(* Logix 5000 AddOnInstructionDefinition export POINT_ADD; software revision 30.00 *)

TYPE POINT :   // A point on an Edwards-curve represented in extended homogeneous coordinates
STRUCT
   X : DINT[22];
   Y : DINT[22];
   Z : DINT[22];
   T : DINT[22];
END_STRUCT
END_TYPE

ADD_ON_INSTRUCTION B256_ADD   (* revision 1.0 20170916, vendor Kenneth A. Fischer *)
// c3=c1+c2 with no reduction
// Revision note:
// Rev1.0: 20170916 - Initial Release
VAR_IN_OUT
   Inp_C1 : DINT[22]; {required}
   Inp_C2 : DINT[22]; {required}
   Out_C3 : DINT[22]; {required}
END_VAR
VAR
   i : INT;
END_VAR

ROUTINE Logic   (* ladder *)
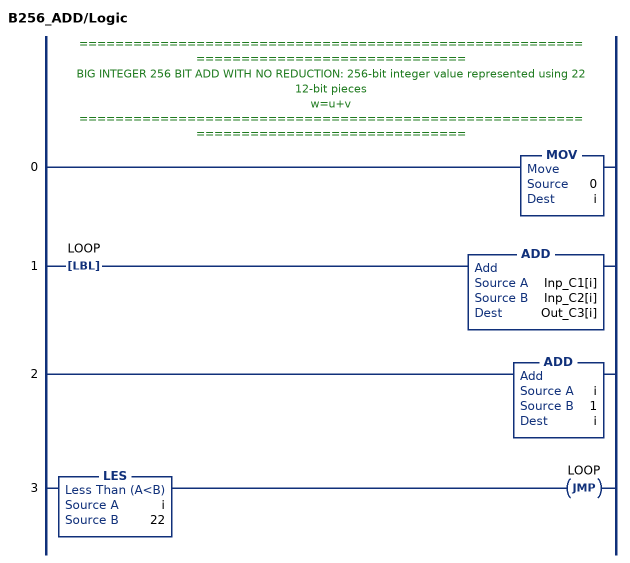
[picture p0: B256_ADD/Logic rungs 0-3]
   // ======================================================================================
   // BIG INTEGER 256 BIT ADD WITH NO REDUCTION: 256-bit integer value represented using 22 12-bit pieces
   // w=u+v
   // ======================================================================================
   0: MOV(0,i);
   1: LBL(LOOP)ADD(Inp_C1[i],Inp_C2[i],Out_C3[i]);
   2: ADD(i,1,i);
   3: LES(i,22)JMP(LOOP);
END_ROUTINE
END_ADD_ON_INSTRUCTION

ADD_ON_INSTRUCTION D_SHR   (* revision 1.0 20170524, vendor Kenneth A. Fischer *)
// DINT bit shift right of the 32-bit argument Inp_A by Inp_B bits with paddding by zeros on the right
// Revision note:
// Rev1.0: 20170524 - Initial Release
VAR_IN_OUT
   Inp_A : DINT; {required}   // 64-bit Integer to be right circular rotated
END_VAR
VAR_INPUT
   Inp_B : INT; {required}   // Number of bits to shift
END_VAR
VAR_IN_OUT
   Out : DINT; {required}   // Result
END_VAR
VAR
   BSR_Cntrl : CONTROL := (LEN := 32);
   ONS : BOOL;
   Source_Bit : BOOL;
   Wrk_InpA : DINT[2];
END_VAR

ROUTINE Logic   (* ladder *)
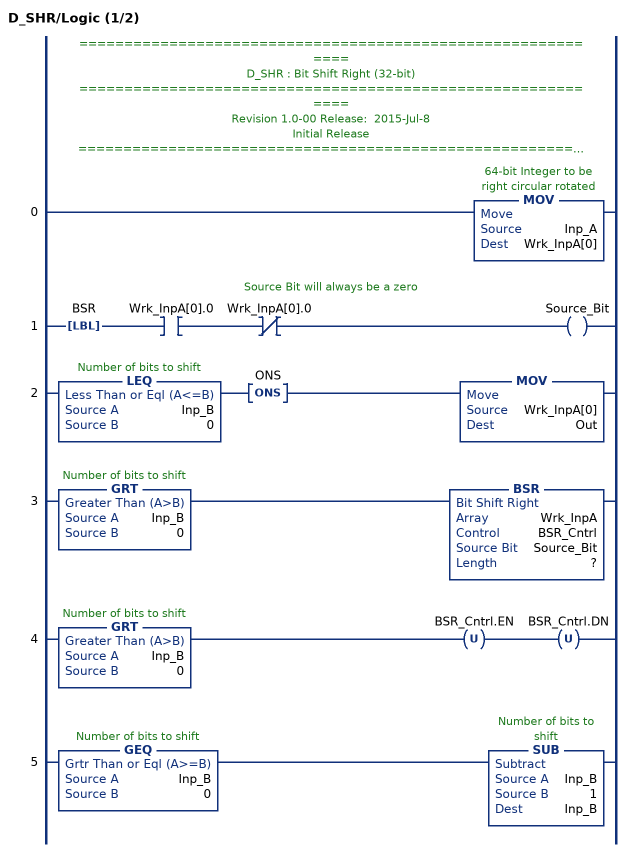
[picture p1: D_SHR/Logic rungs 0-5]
   // ============================================================
   // D_SHR : Bit Shift Right (32-bit)
   // ============================================================
   // Revision 1.0-00 Release:  2015-Jul-8
   // Initial Release
   // ============================================================
   // Performs a right bit shift of the 32-bit argument Inp_A by the
   // number of bits defined in the 16-bit argument Inp_B, with padding by zeros.
   0: MOV(Inp_A,Wrk_InpA[0]);
   // Source Bit will always be a zero
   1: LBL(BSR)XIC(Wrk_InpA[0].0)XIO(Wrk_InpA[0].0)OTE(Source_Bit);
   2: LEQ(Inp_B,0)ONS(ONS)MOV(Wrk_InpA[0],Out);
   3: GRT(Inp_B,0)BSR(Wrk_InpA,BSR_Cntrl,Source_Bit,?);
   4: GRT(Inp_B,0)OTU(BSR_Cntrl.EN)OTU(BSR_Cntrl.DN);
   5: GEQ(Inp_B,0)SUB(Inp_B,1,Inp_B);
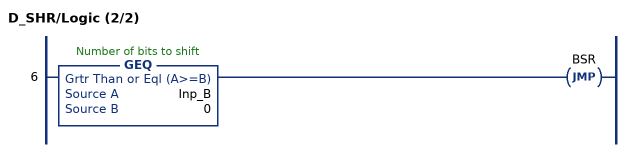
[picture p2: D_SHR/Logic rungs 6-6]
   6: GEQ(Inp_B,0)JMP(BSR);
END_ROUTINE
END_ADD_ON_INSTRUCTION

ADD_ON_INSTRUCTION B256_NRED   (* revision 1.0 20170916, vendor Kenneth A. Fischer *)
// Reduce 256-bit integer stored in 22 pieces by propagating carries
// Revision note:
// Rev1.0: 20170916 - Initial Release
VAR_IN_OUT
   Inp_C : DINT[22]; {required}
END_VAR
VAR
   D_SHR : D_SHR;
   temp : DINT;
   i : INT;
END_VAR

ROUTINE Logic   (* ladder *)
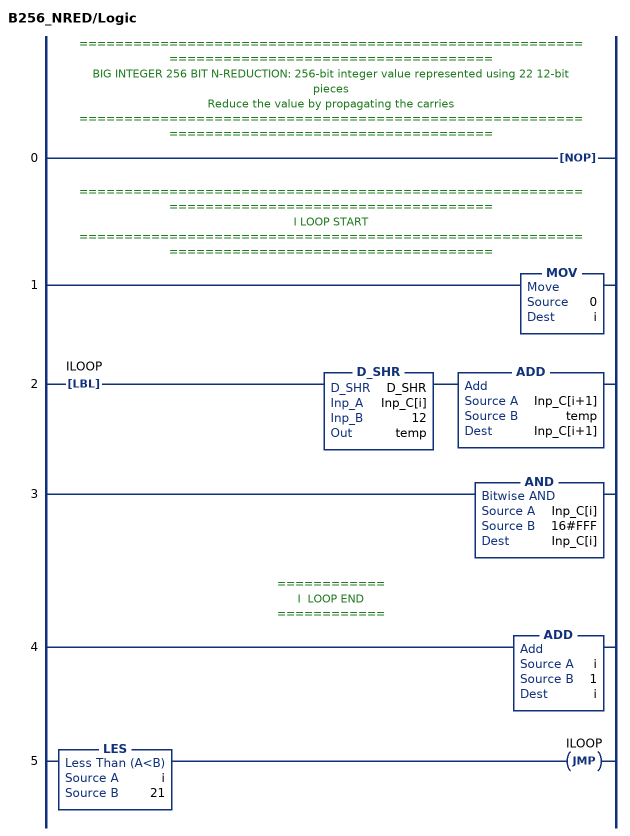
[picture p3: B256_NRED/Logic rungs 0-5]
   // ============================================================================================
   // BIG INTEGER 256 BIT N-REDUCTION: 256-bit integer value represented using 22 12-bit pieces
   // Reduce the value by propagating the carries
   // ============================================================================================
   0: NOP();
   // ============================================================================================
   // I LOOP START
   // ============================================================================================
   1: MOV(0,i);
   2: LBL(ILOOP)D_SHR(D_SHR,Inp_C[i],12,temp)ADD(Inp_C[i+1],temp,Inp_C[i+1]);
   3: AND(Inp_C[i],16#FFF,Inp_C[i]);
   // ============
   // I  LOOP END
   // ============
   4: ADD(i,1,i);
   5: LES(i,21)JMP(ILOOP);
END_ROUTINE
END_ADD_ON_INSTRUCTION

ADD_ON_INSTRUCTION B256_SUB   (* revision 1.0 20170916, vendor Kenneth A. Fischer *)
// c3=c1-c2 with reduction
// Revision note:
// Rev1.0: 20170916 - Initial Release
VAR_IN_OUT
   Inp_C1 : DINT[22]; {required}
   Inp_C2 : DINT[22]; {required}
   Out_C3 : DINT[22]; {required}
END_VAR
VAR
   B256_ADD : B256_ADD;
   B256_NRED : B256_NRED;
   temp : DINT;
   i : INT;
END_VAR

ROUTINE Logic   (* ladder *)
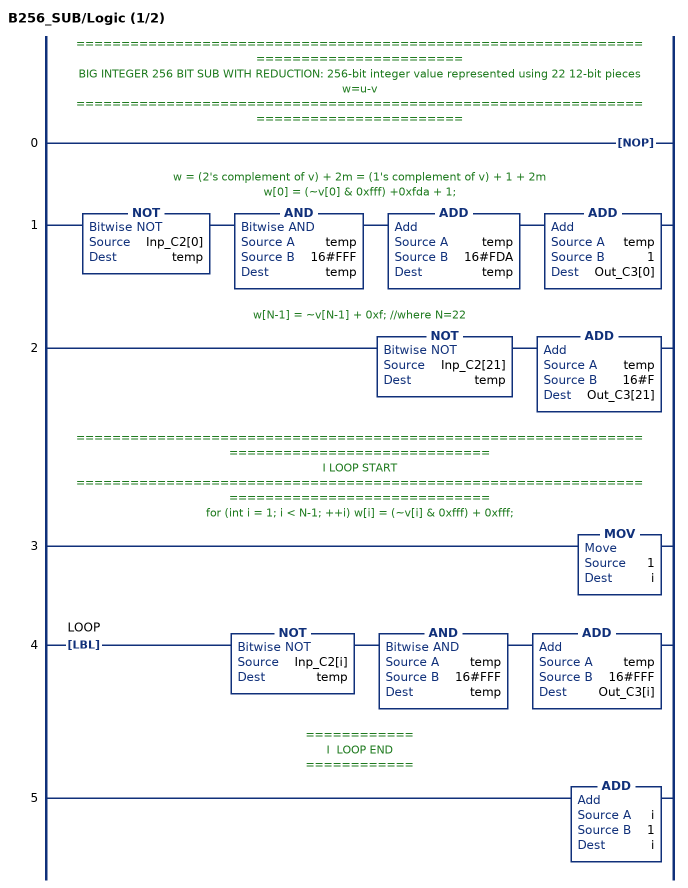
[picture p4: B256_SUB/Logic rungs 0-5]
   // ======================================================================================
   // BIG INTEGER 256 BIT SUB WITH REDUCTION: 256-bit integer value represented using 22 12-bit pieces
   //  w=u-v
   // ======================================================================================
   0: NOP();
   // w = (2's complement of v) + 2m = (1's complement of v) + 1 + 2m
   // w[0] = (~v[0] & 0xfff) +0xfda + 1;
   1: NOT(Inp_C2[0],temp)AND(temp,16#FFF,temp)ADD(temp,16#FDA,temp)ADD(temp,1,Out_C3[0]);
   // w[N-1] = ~v[N-1] + 0xf; //where N=22
   2: NOT(Inp_C2[21],temp)ADD(temp,16#F,Out_C3[21]);
   // ============================================================================================
   // I LOOP START
   // ============================================================================================
   // for (int i = 1; i < N-1; ++i) w[i] = (~v[i] & 0xfff) + 0xfff;
   3: MOV(1,i);
   4: LBL(LOOP)NOT(Inp_C2[i],temp)AND(temp,16#FFF,temp)ADD(temp,16#FFF,Out_C3[i]);
   // ============
   // I  LOOP END
   // ============
   5: ADD(i,1,i);
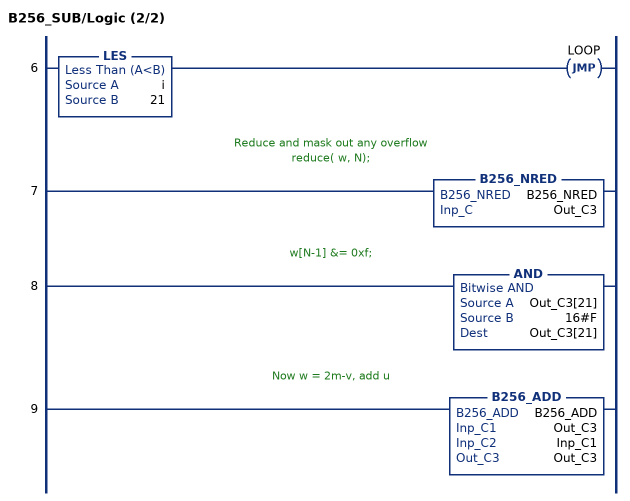
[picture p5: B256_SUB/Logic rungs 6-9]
   6: LES(i,21)JMP(LOOP);
   // Reduce and mask out any overflow
   // reduce( w, N);
   7: B256_NRED(B256_NRED,Out_C3);
   // w[N-1] &= 0xf;
   8: AND(Out_C3[21],16#F,Out_C3[21]);
   // Now w = 2m-v, add u
   9: B256_ADD(B256_ADD,Out_C3,Inp_C1,Out_C3);
END_ROUTINE
END_ADD_ON_INSTRUCTION

ADD_ON_INSTRUCTION B256_FRED   (* revision 1.0 20170916, vendor Kenneth A. Fischer *)
// fast_reduce:  reduce by propagating the carries starting at a particular offset and stoping once the carry becomes zero
// Revision note:
// Rev1.0: 20170916 - Initial Release
VAR_IN_OUT
   Inp_C : DINT[22]; {required}
END_VAR
VAR_INPUT
   Inp_offset : INT; {required}
END_VAR
VAR
   i : INT;
   carry : DINT;
   D_SHR : D_SHR;
END_VAR

ROUTINE Logic   (* ladder *)
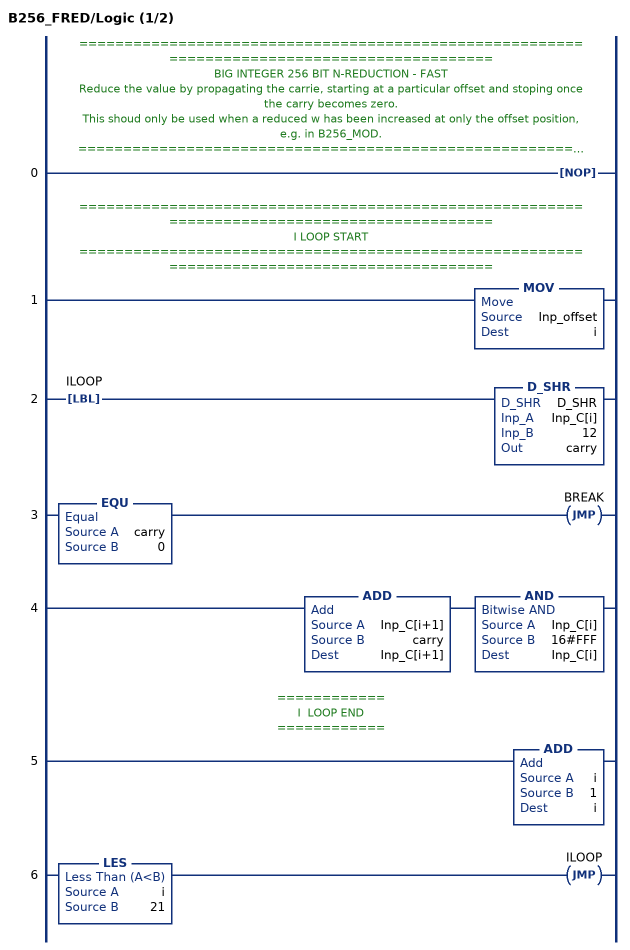
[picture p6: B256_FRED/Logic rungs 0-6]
   // ============================================================================================
   // BIG INTEGER 256 BIT N-REDUCTION - FAST
   // Reduce the value by propagating the carrie, starting at a particular offset and stoping once the carry becomes zero.
   // This shoud only be used when a reduced w has been increased at only the offset position, e.g. in B256_MOD.
   // ============================================================================================
   0: NOP();
   // ============================================================================================
   // I LOOP START
   // ============================================================================================
   1: MOV(Inp_offset,i);
   2: LBL(ILOOP)D_SHR(D_SHR,Inp_C[i],12,carry);
   3: EQU(carry,0)JMP(BREAK);
   4: ADD(Inp_C[i+1],carry,Inp_C[i+1])AND(Inp_C[i],16#FFF,Inp_C[i]);
   // ============
   // I  LOOP END
   // ============
   5: ADD(i,1,i);
   6: LES(i,21)JMP(ILOOP);
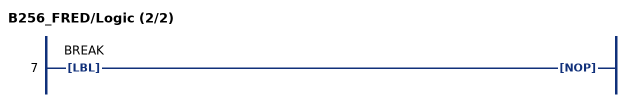
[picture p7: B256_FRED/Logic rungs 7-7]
   7: LBL(BREAK)NOP();
END_ROUTINE
END_ADD_ON_INSTRUCTION

ADD_ON_INSTRUCTION D_SHL   (* revision 1.0 20170524, vendor Kenneth A. Fischer *)
// DINT bit shift left of the 32-bit argument Inp_A by Inp_B bits with paddding by zeros on the right
// Revision note:
// Rev1.0: 20170524 - Initial Release
VAR_IN_OUT
   Inp_A : DINT; {required}   // 64-bit Integer to be right circular rotated
END_VAR
VAR_INPUT
   Inp_B : INT; {required}   // Number of bits to shift
END_VAR
VAR_IN_OUT
   Out : DINT; {required}   // Result
END_VAR
VAR
   Wrk_InpA : DINT[2];
   Source_Bit : BOOL;
   ONS : BOOL;
   BSL_Cntrl : CONTROL := (LEN := 32);
END_VAR

ROUTINE Logic   (* ladder *)
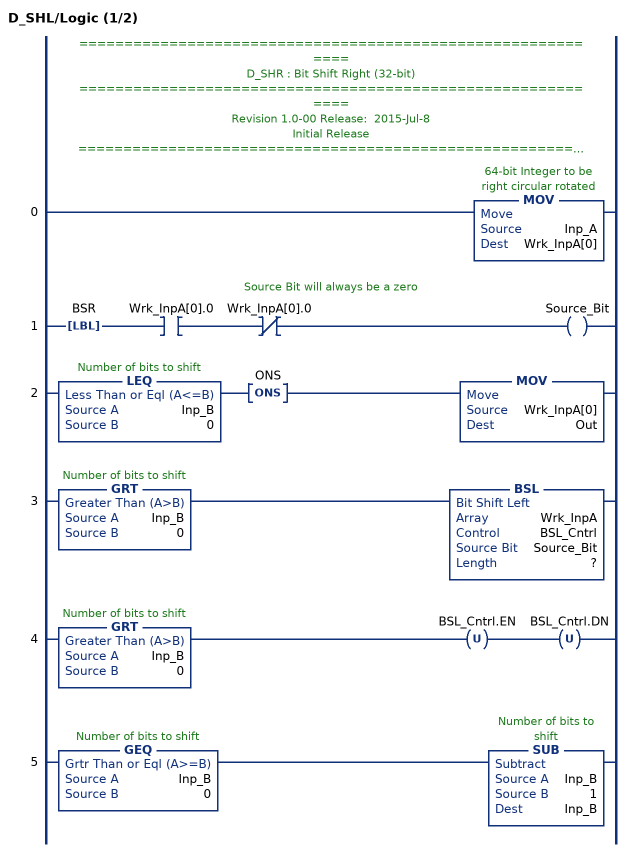
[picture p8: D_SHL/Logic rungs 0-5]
   // ============================================================
   // D_SHR : Bit Shift Right (32-bit)
   // ============================================================
   // Revision 1.0-00 Release:  2015-Jul-8
   // Initial Release
   // ============================================================
   // Performs a left bit shift of the 32-bit argument Inp_A by the
   // number of bits defined in the 16-bit argument Inp_B, with padding by zeros.
   0: MOV(Inp_A,Wrk_InpA[0]);
   // Source Bit will always be a zero
   1: LBL(BSR)XIC(Wrk_InpA[0].0)XIO(Wrk_InpA[0].0)OTE(Source_Bit);
   2: LEQ(Inp_B,0)ONS(ONS)MOV(Wrk_InpA[0],Out);
   3: GRT(Inp_B,0)BSL(Wrk_InpA,BSL_Cntrl,Source_Bit,?);
   4: GRT(Inp_B,0)OTU(BSL_Cntrl.EN)OTU(BSL_Cntrl.DN);
   5: GEQ(Inp_B,0)SUB(Inp_B,1,Inp_B);
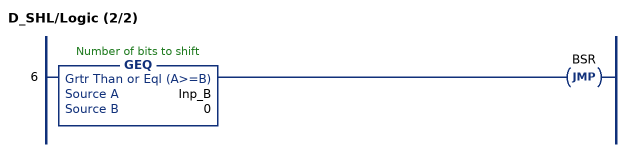
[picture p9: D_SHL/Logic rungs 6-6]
   6: GEQ(Inp_B,0)JMP(BSR);
END_ROUTINE
END_ADD_ON_INSTRUCTION

ADD_ON_INSTRUCTION B256_MOD   (* revision 1.0 20170916, vendor Kenneth A. Fischer *)
// c = d mod (2^255 - 19)
// Revision note:
// Rev1.0: 20170916 - Initial Release
VAR_IN_OUT
   Inp_D : DINT[43]; {required}
   Out_C : DINT[22]; {required}
END_VAR
VAR
   B256_NRED : B256_NRED;
   D_SHL : D_SHL;
   D_SHR : D_SHR;
   i : INT;
   t : DINT;
   temp : DINT;
   temp2 : DINT;
   B256_FRED : B256_FRED;
   offset : DINT;
END_VAR

ROUTINE Logic   (* ladder *)
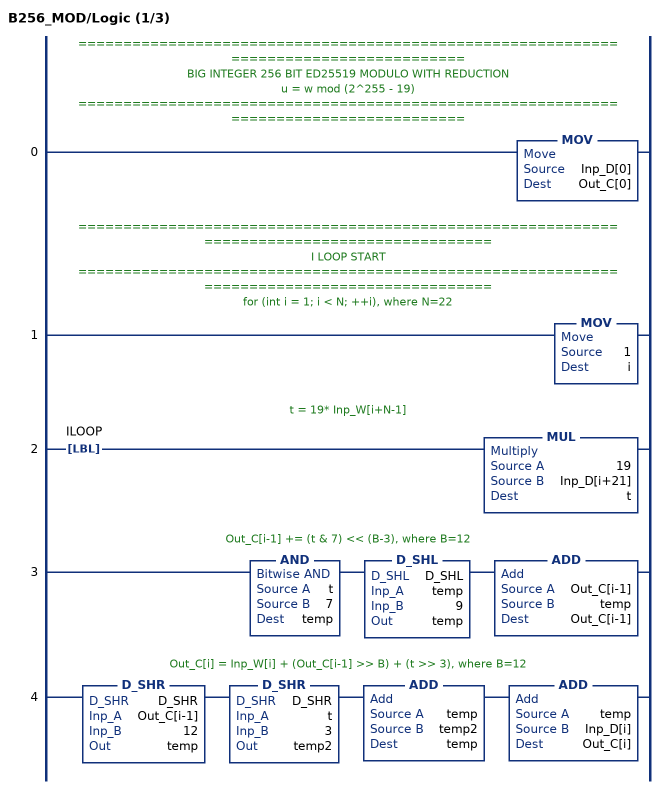
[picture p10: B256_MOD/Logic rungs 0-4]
   // ======================================================================================
   // BIG INTEGER 256 BIT ED25519 MODULO WITH REDUCTION
   //  u = w mod (2^255 - 19)
   // ======================================================================================
   0: MOV(Inp_D[0],Out_C[0]);
   // ============================================================================================
   // I LOOP START
   // ============================================================================================
   // for (int i = 1; i < N; ++i), where N=22
   1: MOV(1,i);
   // t = 19* Inp_W[i+N-1]
   2: LBL(ILOOP)MUL(19,Inp_D[i+21],t);
   // Out_C[i-1] += (t & 7) << (B-3), where B=12
   3: AND(t,7,temp)D_SHL(D_SHL,temp,9,temp)ADD(Out_C[i-1],temp,Out_C[i-1]);
   // Out_C[i] = Inp_W[i] + (Out_C[i-1] >> B) + (t >> 3), where B=12
   4: D_SHR(D_SHR,Out_C[i-1],12,temp)D_SHR(D_SHR,t,3,temp2)ADD(temp,temp2,temp)ADD(temp,Inp_D[i],Out_C[i]);
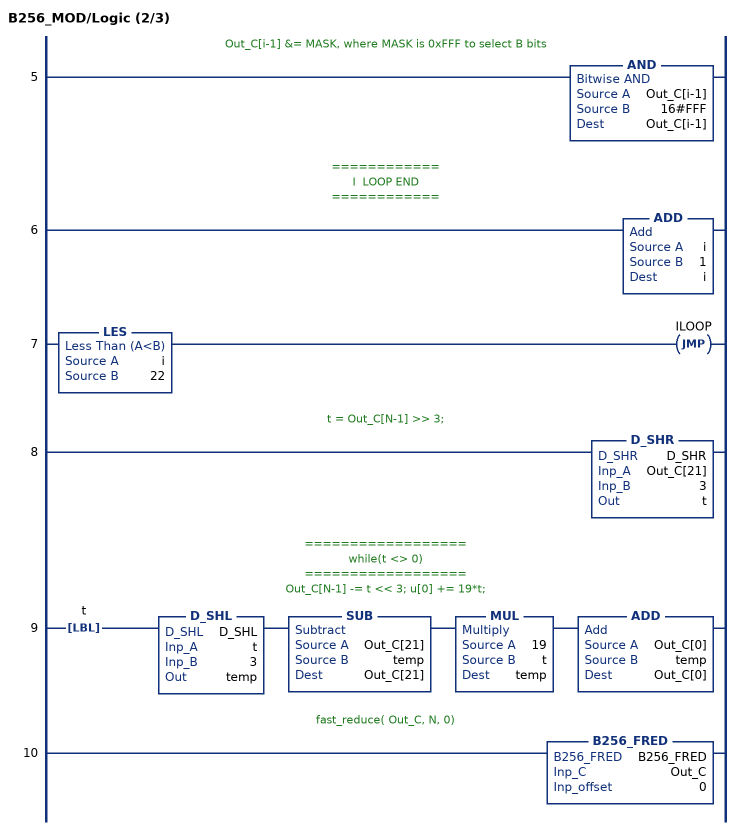
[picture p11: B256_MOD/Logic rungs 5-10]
   // Out_C[i-1] &= MASK, where MASK is 0xFFF to select B bits
   5: AND(Out_C[i-1],16#FFF,Out_C[i-1]);
   // ============
   // I  LOOP END
   // ============
   6: ADD(i,1,i);
   7: LES(i,22)JMP(ILOOP);
   // t = Out_C[N-1] >> 3;
   8: D_SHR(D_SHR,Out_C[21],3,t);
   // ==================
   // while(t <> 0)
   // ==================
   // Out_C[N-1] -= t << 3; u[0] += 19*t;
   9: LBL(t)D_SHL(D_SHL,t,3,temp)SUB(Out_C[21],temp,Out_C[21])MUL(19,t,temp)ADD(Out_C[0],temp,Out_C[0]);
   // fast_reduce( Out_C, N, 0)
   10: B256_FRED(B256_FRED,Out_C,0);
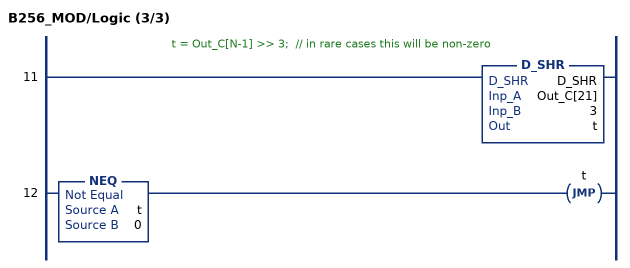
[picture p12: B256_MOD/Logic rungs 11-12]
   // t = Out_C[N-1] >> 3;  // in rare cases this will be non-zero
   11: D_SHR(D_SHR,Out_C[21],3,t);
   12: NEQ(t,0)JMP(t);
END_ROUTINE
END_ADD_ON_INSTRUCTION

ADD_ON_INSTRUCTION B256_NNRED   (* revision 1.0 20170916, vendor Kenneth A. Fischer *)
// Reduce 256-bit integer stored in 43 pieces by propagating carries
// Revision note:
// Rev1.0: 20170916 - Initial Release
VAR_IN_OUT
   Inp_D : DINT[43]; {required}
END_VAR
VAR
   temp : DINT;
   i : INT;
   D_SHR : D_SHR;
END_VAR

ROUTINE Logic   (* ladder *)
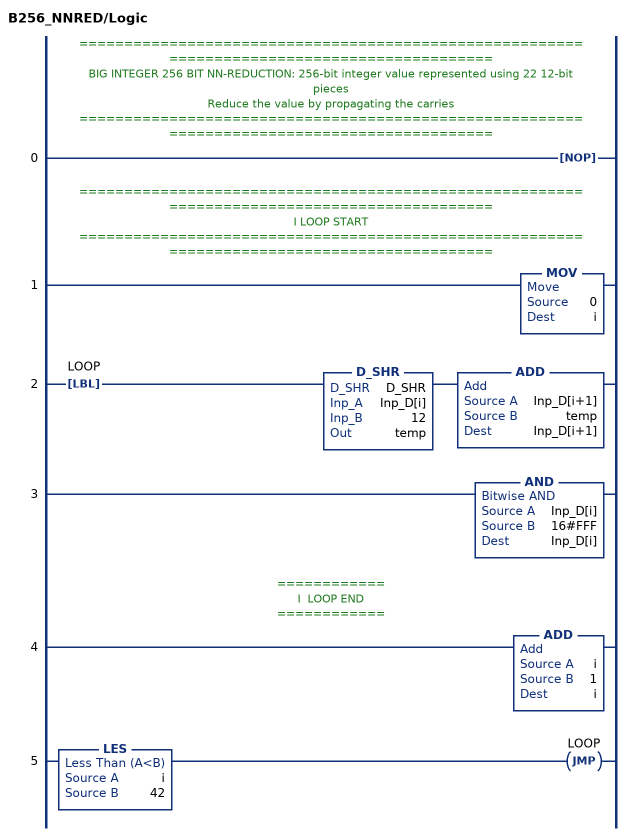
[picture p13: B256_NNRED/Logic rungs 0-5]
   // ============================================================================================
   // BIG INTEGER 256 BIT NN-REDUCTION: 256-bit integer value represented using 22 12-bit pieces
   // Reduce the value by propagating the carries
   // ============================================================================================
   0: NOP();
   // ============================================================================================
   // I LOOP START
   // ============================================================================================
   1: MOV(0,i);
   2: LBL(LOOP)D_SHR(D_SHR,Inp_D[i],12,temp)ADD(Inp_D[i+1],temp,Inp_D[i+1]);
   3: AND(Inp_D[i],16#FFF,Inp_D[i]);
   // ============
   // I  LOOP END
   // ============
   4: ADD(i,1,i);
   5: LES(i,42)JMP(LOOP);
END_ROUTINE
END_ADD_ON_INSTRUCTION

ADD_ON_INSTRUCTION B256_MUL   (* revision 1.0 20170916, vendor Kenneth A. Fischer *)
// c3 = c1*c2 with reduction and mod
// Revision note:
// Rev1.0: 20170916 - Initial Release
VAR_IN_OUT
   Temp_D : DINT[43]; {required}
   Inp_C1 : DINT[22]; {required}
   Inp_C2 : DINT[22]; {required}
   Out_C3 : DINT[22]; {required}
END_VAR
VAR
   B256_MOD : B256_MOD;
   B256_NNRED : B256_NNRED;
   i : INT;
   j : INT;
   mul_temp : DINT;
END_VAR

ROUTINE Logic   (* ladder *)
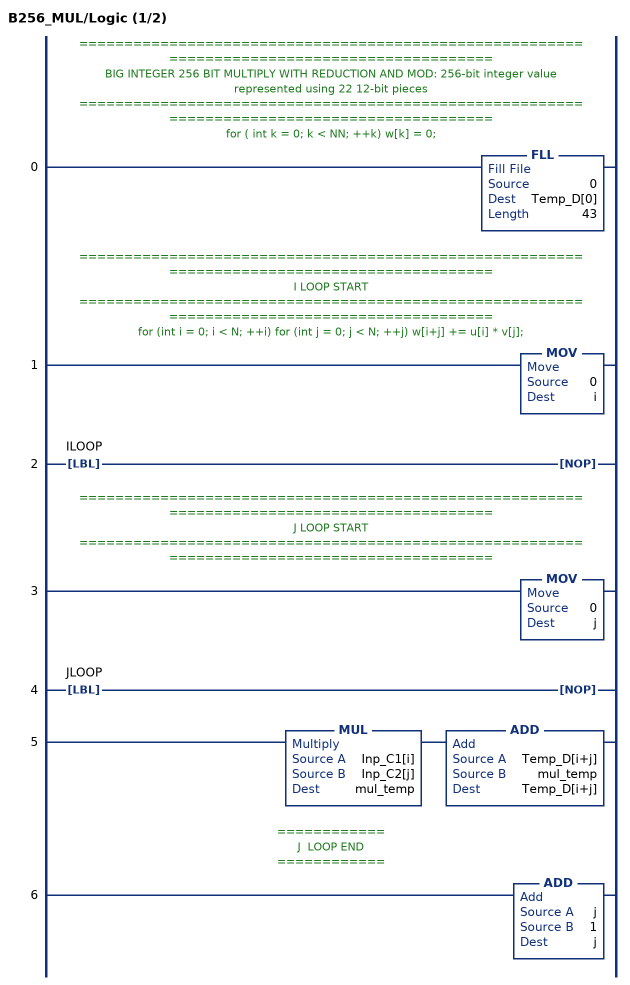
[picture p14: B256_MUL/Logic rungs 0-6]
   // ============================================================================================
   // BIG INTEGER 256 BIT MULTIPLY WITH REDUCTION AND MOD: 256-bit integer value represented using 22 12-bit pieces
   // ============================================================================================
   // for ( int k = 0; k < NN; ++k) w[k] = 0;
   0: FLL(0,Temp_D[0],43);
   // ============================================================================================
   // I LOOP START
   // ============================================================================================
   // for (int i = 0; i < N; ++i) for (int j = 0; j < N; ++j) w[i+j] += u[i] * v[j];
   1: MOV(0,i);
   2: LBL(ILOOP)NOP();
   // ============================================================================================
   // J LOOP START
   // ============================================================================================
   3: MOV(0,j);
   4: LBL(JLOOP)NOP();
   5: MUL(Inp_C1[i],Inp_C2[j],mul_temp)ADD(Temp_D[i+j],mul_temp,Temp_D[i+j]);
   // ============
   // J  LOOP END
   // ============
   6: ADD(j,1,j);
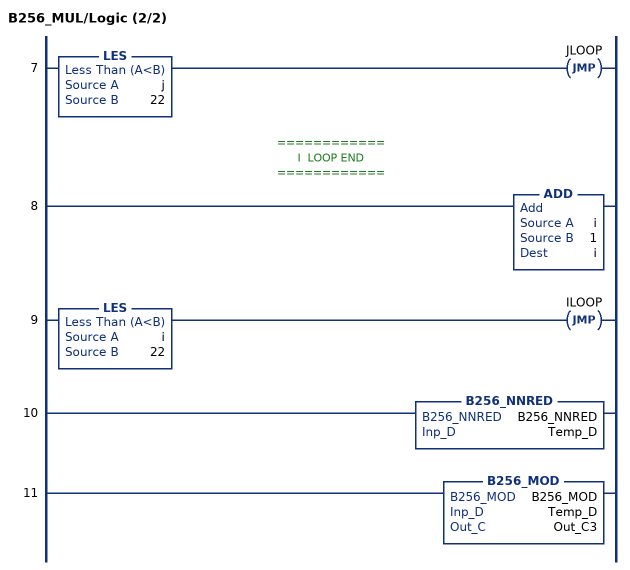
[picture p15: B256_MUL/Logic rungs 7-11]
   7: LES(j,22)JMP(JLOOP);
   // ============
   // I  LOOP END
   // ============
   8: ADD(i,1,i);
   9: LES(i,22)JMP(ILOOP);
   10: B256_NNRED(B256_NNRED,Temp_D);
   11: B256_MOD(B256_MOD,Temp_D,Out_C3);
END_ROUTINE
END_ADD_ON_INSTRUCTION

ADD_ON_INSTRUCTION B256_MUL2   (* revision 1.0 20170916, vendor Kenneth A. Fischer *)
// c3= 2*c1*c2 with reduction and mod
// Revision note:
// Rev1.0: 20170916 - Initial Release
VAR_IN_OUT
   Temp_D : DINT[43]; {required}
   Inp_C1 : DINT[22]; {required}
   Inp_C2 : DINT[22]; {required}
   Out_C3 : DINT[22]; {required}
END_VAR
VAR
   B256_NNRED : B256_NNRED;
   i : INT;
   j : INT;
   mul_temp : DINT;
   B256_MOD : B256_MOD;
   t : DINT;
END_VAR

ROUTINE Logic   (* ladder *)
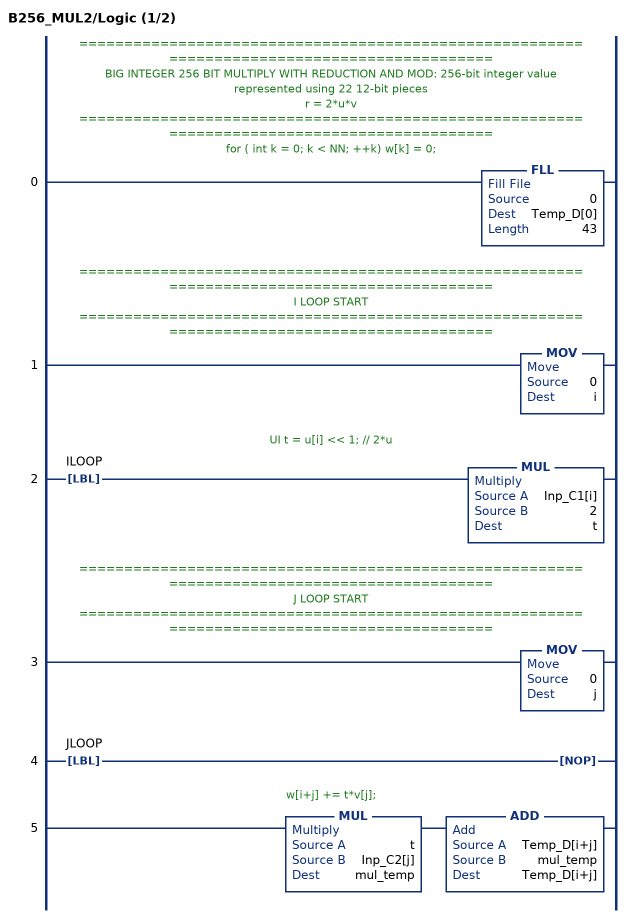
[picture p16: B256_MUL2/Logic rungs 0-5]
   // ============================================================================================
   // BIG INTEGER 256 BIT MULTIPLY WITH REDUCTION AND MOD: 256-bit integer value represented using 22 12-bit pieces
   // r = 2*u*v
   // ============================================================================================
   // for ( int k = 0; k < NN; ++k) w[k] = 0;
   0: FLL(0,Temp_D[0],43);
   // ============================================================================================
   // I LOOP START
   // ============================================================================================
   1: MOV(0,i);
   // UI t = u[i] << 1; // 2*u
   2: LBL(ILOOP)MUL(Inp_C1[i],2,t);
   // ============================================================================================
   // J LOOP START
   // ============================================================================================
   3: MOV(0,j);
   4: LBL(JLOOP)NOP();
   // w[i+j] += t*v[j];
   5: MUL(t,Inp_C2[j],mul_temp)ADD(Temp_D[i+j],mul_temp,Temp_D[i+j]);
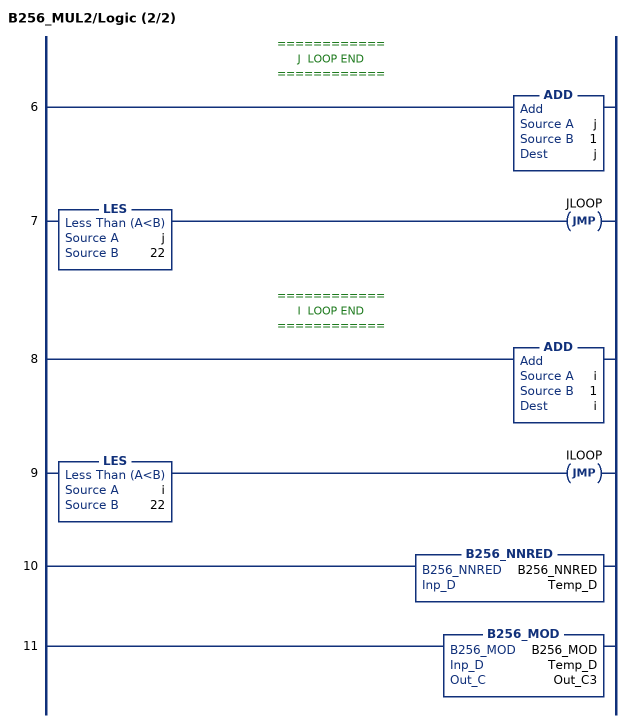
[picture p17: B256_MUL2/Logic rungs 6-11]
   // ============
   // J  LOOP END
   // ============
   6: ADD(j,1,j);
   7: LES(j,22)JMP(JLOOP);
   // ============
   // I  LOOP END
   // ============
   8: ADD(i,1,i);
   9: LES(i,22)JMP(ILOOP);
   10: B256_NNRED(B256_NNRED,Temp_D);
   11: B256_MOD(B256_MOD,Temp_D,Out_C3);
END_ROUTINE
END_ADD_ON_INSTRUCTION

ADD_ON_INSTRUCTION POINT_ADD   (* revision 1.0 20170916, vendor Kenneth A. Fischer *)
// Point Add:
// p3 = p1 + p2
// Requires POINT UDT
// Revision note:
// Rev1.0: 20170916 - Initial Release
VAR_IN_OUT
   Temp_C1 : DINT[22]; {required}   // A
   Temp_C2 : DINT[22]; {required}   // B
   Temp_C3 : DINT[22]; {required}   // C
   Temp_C4 : DINT[22]; {required}   // D
   Temp_C5 : DINT[22]; {required}   // E
   Temp_C6 : DINT[22]; {required}   // F
   Temp_C7 : DINT[22]; {required}   // G
   Temp_C8 : DINT[22]; {required}   // H
   Temp_C9 : DINT[22]; {required}   // R
   Temp_C10 : DINT[22]; {required}   // S
   Temp_D : DINT[43]; {required}   // W
   Inp_P1 : POINT; {required}
   Inp_P2 : POINT; {required}
   Out_P3 : POINT; {required}
END_VAR
VAR
   B256_SUB : B256_SUB;
   B256_ADD : B256_ADD;
   B256_MUL : B256_MUL;
   B256_MUL2 : B256_MUL2;
END_VAR

ROUTINE Logic   (* ladder *)
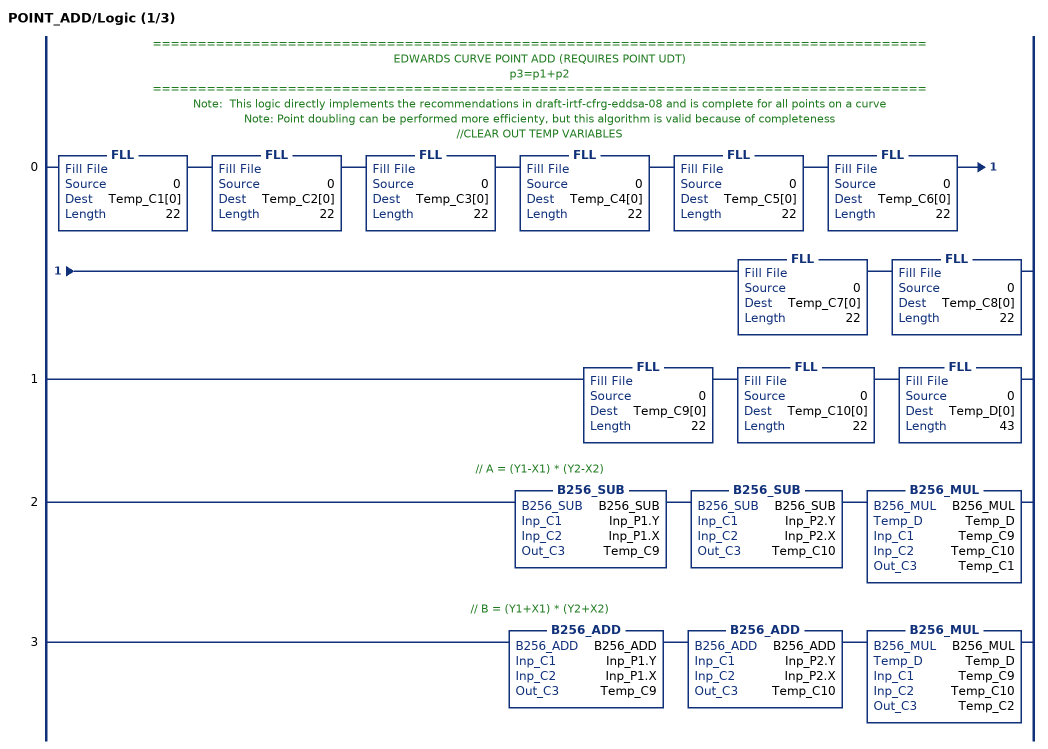
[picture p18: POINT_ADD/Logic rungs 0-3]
   // ======================================================================================
   // EDWARDS CURVE POINT ADD (REQUIRES POINT UDT)
   // p3=p1+p2
   // ======================================================================================
   // Note:  This logic directly implements the recommendations in draft-irtf-cfrg-eddsa-08 and is complete for all points on a curve
   // Note: Point doubling can be performed more efficienty, but this algorithm is valid because of completeness
   // //CLEAR OUT TEMP VARIABLES
   0: FLL(0,Temp_C1[0],22)FLL(0,Temp_C2[0],22)FLL(0,Temp_C3[0],22)FLL(0,Temp_C4[0],22)FLL(0,Temp_C5[0],22)FLL(0,Temp_C6[0],22)FLL(0,Temp_C7[0],22)FLL(0,Temp_C8[0],22);
   1: FLL(0,Temp_C9[0],22)FLL(0,Temp_C10[0],22)FLL(0,Temp_D[0],43);
   // // A = (Y1-X1) * (Y2-X2)
   2: B256_SUB(B256_SUB,Inp_P1.Y,Inp_P1.X,Temp_C9)B256_SUB(B256_SUB,Inp_P2.Y,Inp_P2.X,Temp_C10)B256_MUL(B256_MUL,Temp_D,Temp_C9,Temp_C10,Temp_C1);
   // // B = (Y1+X1) * (Y2+X2)
   3: B256_ADD(B256_ADD,Inp_P1.Y,Inp_P1.X,Temp_C9)B256_ADD(B256_ADD,Inp_P2.Y,Inp_P2.X,Temp_C10)B256_MUL(B256_MUL,Temp_D,Temp_C9,Temp_C10,Temp_C2);
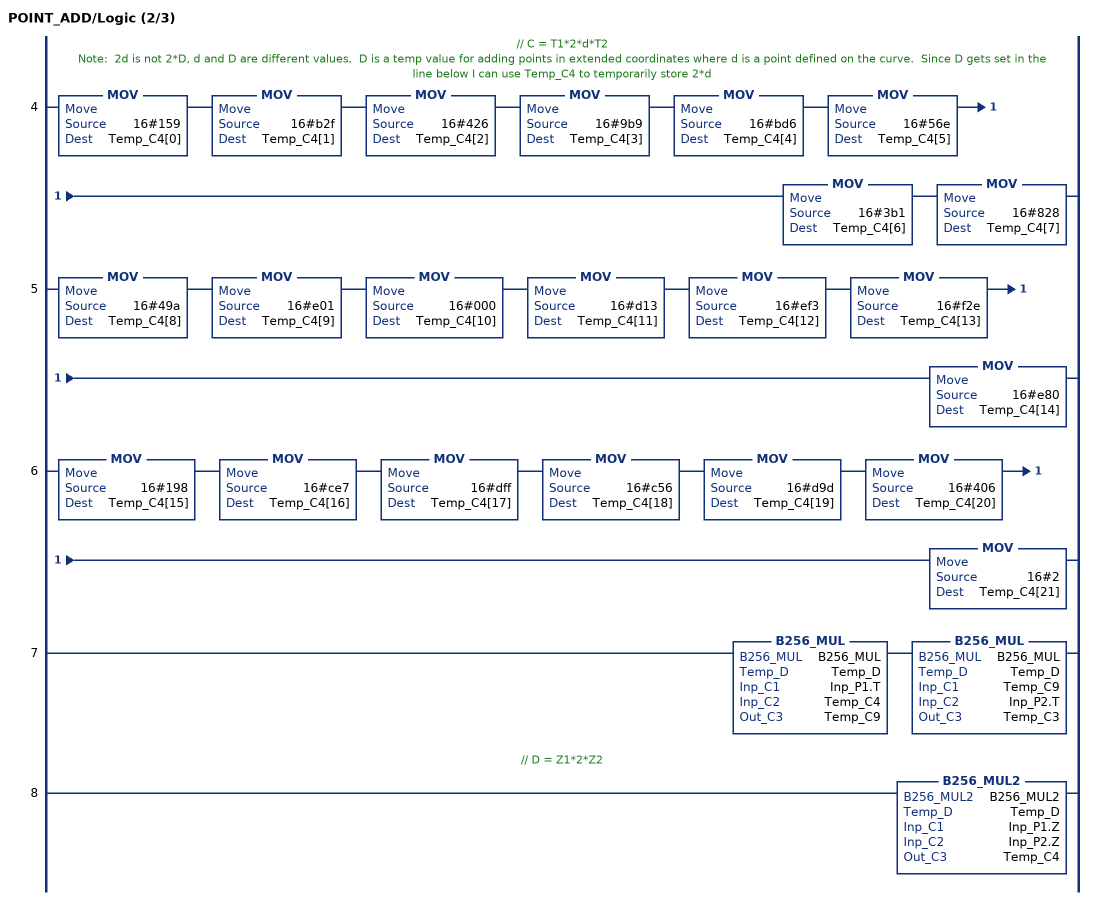
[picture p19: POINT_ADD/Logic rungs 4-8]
   // // C = T1*2*d*T2
   // Note:  2d is not 2*D, d and D are different values.  D is a temp value for adding points in extended coordinates where d is a point defined on the curve.  Since D gets set in the line below I can use Temp_C4 to temporarily store 2*d
   4: MOV(16#159,Temp_C4[0])MOV(16#b2f,Temp_C4[1])MOV(16#426,Temp_C4[2])MOV(16#9b9,Temp_C4[3])MOV(16#bd6,Temp_C4[4])MOV(16#56e,Temp_C4[5])MOV(16#3b1,Temp_C4[6])MOV(16#828,Temp_C4[7]);
   5: MOV(16#49a,Temp_C4[8])MOV(16#e01,Temp_C4[9])MOV(16#000,Temp_C4[10])MOV(16#d13,Temp_C4[11])MOV(16#ef3,Temp_C4[12])MOV(16#f2e,Temp_C4[13])MOV(16#e80,Temp_C4[14]);
   6: MOV(16#198,Temp_C4[15])MOV(16#ce7,Temp_C4[16])MOV(16#dff,Temp_C4[17])MOV(16#c56,Temp_C4[18])MOV(16#d9d,Temp_C4[19])MOV(16#406,Temp_C4[20])MOV(16#2,Temp_C4[21]);
   7: B256_MUL(B256_MUL,Temp_D,Inp_P1.T,Temp_C4,Temp_C9)B256_MUL(B256_MUL,Temp_D,Temp_C9,Inp_P2.T,Temp_C3);
   // // D = Z1*2*Z2
   8: B256_MUL2(B256_MUL2,Temp_D,Inp_P1.Z,Inp_P2.Z,Temp_C4);
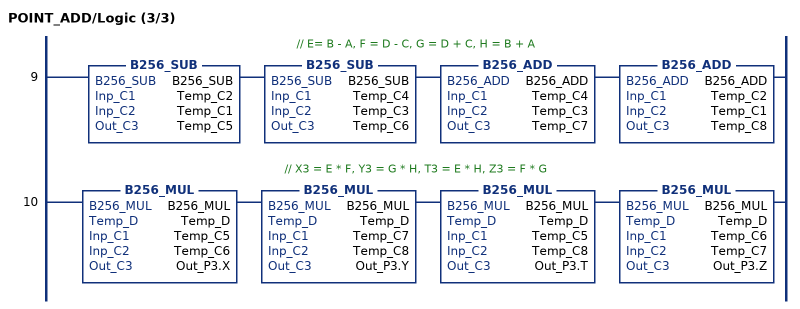
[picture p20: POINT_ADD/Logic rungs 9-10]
   // // E= B - A, F = D - C, G = D + C, H = B + A
   9: B256_SUB(B256_SUB,Temp_C2,Temp_C1,Temp_C5)B256_SUB(B256_SUB,Temp_C4,Temp_C3,Temp_C6)B256_ADD(B256_ADD,Temp_C4,Temp_C3,Temp_C7)B256_ADD(B256_ADD,Temp_C2,Temp_C1,Temp_C8);
   // // X3 = E * F, Y3 = G * H, T3 = E * H, Z3 = F * G
   10: B256_MUL(B256_MUL,Temp_D,Temp_C5,Temp_C6,Out_P3.X)B256_MUL(B256_MUL,Temp_D,Temp_C7,Temp_C8,Out_P3.Y)B256_MUL(B256_MUL,Temp_D,Temp_C5,Temp_C8,Out_P3.T)B256_MUL(B256_MUL,Temp_D,Temp_C6,Temp_C7,Out_P3.Z);
END_ROUTINE
END_ADD_ON_INSTRUCTION
